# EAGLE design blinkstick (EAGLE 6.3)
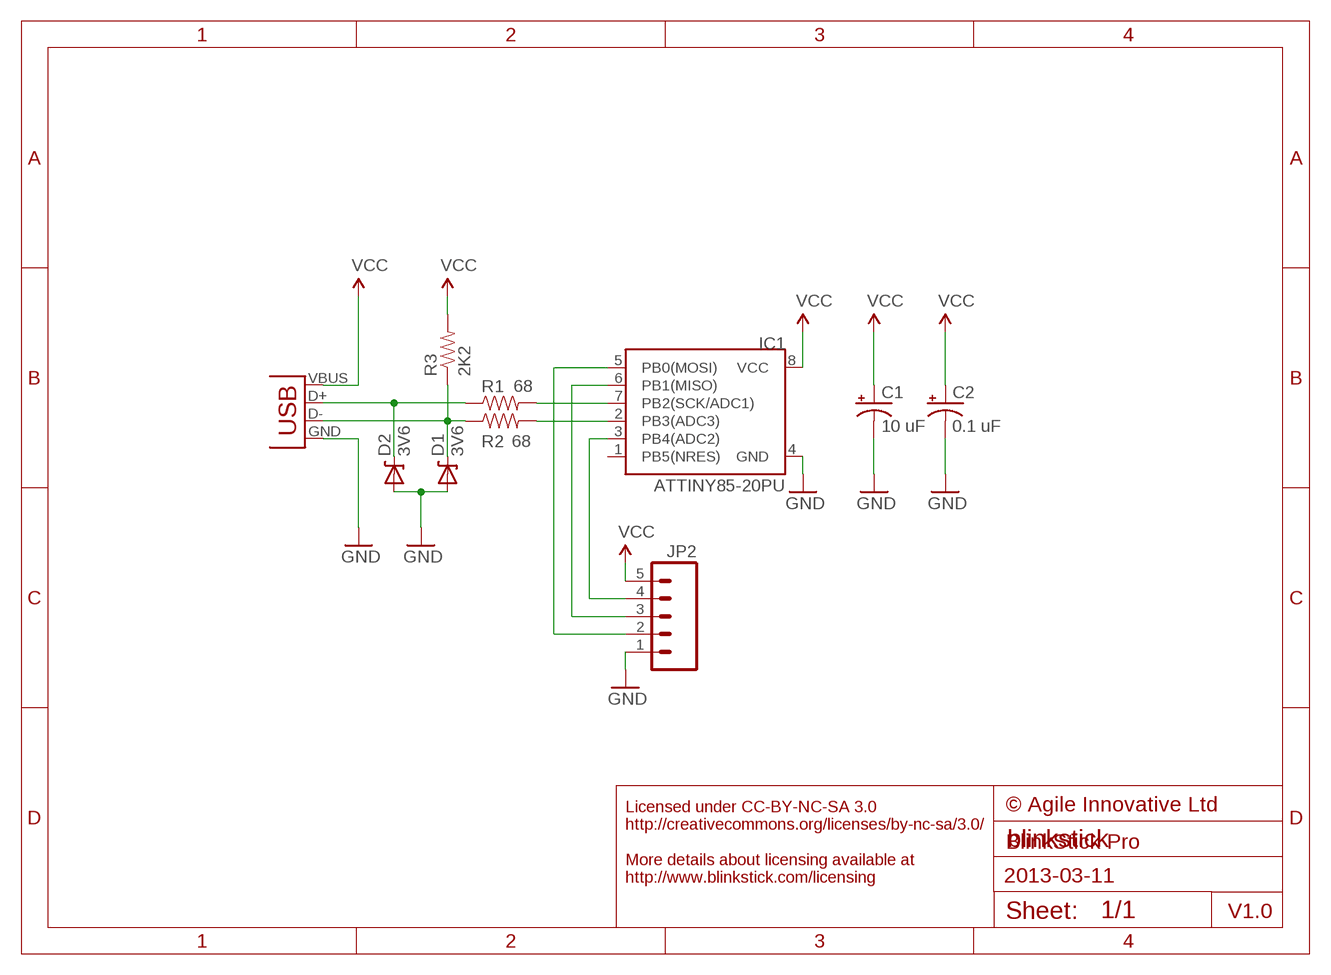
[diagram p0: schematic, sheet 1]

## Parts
C1  10 uF  CAP_POLPTH2  [CPOL-RADIAL-10UF-25V]
C2  0.1 uF  CAP_POLPTH2-1  [CPOL-PTH-10UF-25V]
D1  3V6  DIODE-ZENERPTH  [DIODE-ZENER]
D2  3V6  DIODE-ZENERPTH  [DIODE-ZENER]
IC1  ATTINY85-20PU  ATTINY45TINY45-20-DIP  [DIP08]
JP1  USB-A-H  [USB-A-H]
JP2  M05PTH  [1X05]
R1  68  RESISTORPTH-1/4W  [AXIAL-0.4]
R2  68  RESISTORPTH-1/4W  [AXIAL-0.4]
R3  2K2  RESISTORPTH-1/4W  [AXIAL-0.4]

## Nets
GND: C1.2(-) C2.2(-) D1.P$2(A) D2.P$2(A) IC1.4(GND) JP1.GND(VBUS) JP2.1
N$1: D2.P$1(C) JP1.D+(D-) R1.P$1
N$2: IC1.7(PB2(SCK/ADC1)) R1.P$2
N$3: IC1.2(PB3(ADC3)) R2.P$2
N$4: D1.P$1(C) JP1.D-(D+) R2.P$1 R3.P$1
N$5: IC1.3(PB4(ADC2)) JP2.4
N$6: IC1.6(PB1(MISO)) JP2.3
N$7: IC1.5(PB0(MOSI)) JP2.2
VCC: C1.1(+) C2.1(+) IC1.8(VCC) JP1.VBUS(GND) JP2.5 R3.P$2
Unconnected: IC1.1(PB5(NRES))

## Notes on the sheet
- © Agile Innovative Ltd
- BlinkStick Pro
- Licensed under CC-BY-NC-SA 3.0
  http://creativecommons.org/licenses/by-nc-sa/3.0/
  
  More details about licensing available at
  http://www.blinkstick.com/licensing
- 2013-03-11
- V1.0

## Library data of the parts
C1 = SparkFun-Capacitors:CAP_POL: Capacitor Polarized
C2 = generic:CAP_POL: Capacitor Polarized
D1 D2 = generic:DIODE-ZENER: Zener Diode
IC1 = SparkFun-DigitalIC big pads:ATTINY45: Atmel 8-pin 2/4/8kB flash uC; PROD_ID: IC-09439; VALUE: TINY45-20-DIP
JP1 = generic:USB: USB Connectors USB-B-PTH is fully proven SKU : PRT-00139/CONN-08278 USB-miniB is fully proven SKU : PRT-00587 USB-A-PCB is untested. USB-A-H is throughly reviewed, but untested. Spark Fun Electronics SKU : PRT-00437 USB-B-SMT is throughly reviewed, but untested. Needs silkscreen touching up.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
JP2 = SparkFun-Connectors:M05: Header 5 Standard 5-pin 0.1" header. Use with straight break away headers (SKU : PRT-00116), right angle break away headers (PRT-00553), swiss pins (PRT-00743), machine pins (PRT-00117), and female headers (PRT-00115). Molex polarized connector foot print use with SKU : PRT-08230 with associated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
R1-R3 = SparkFun-Passives:RESISTOR: Resistor

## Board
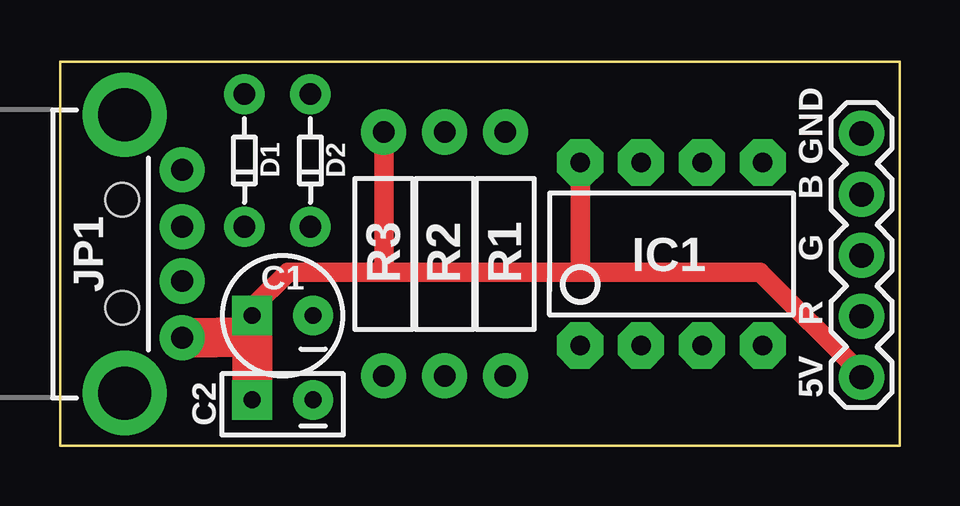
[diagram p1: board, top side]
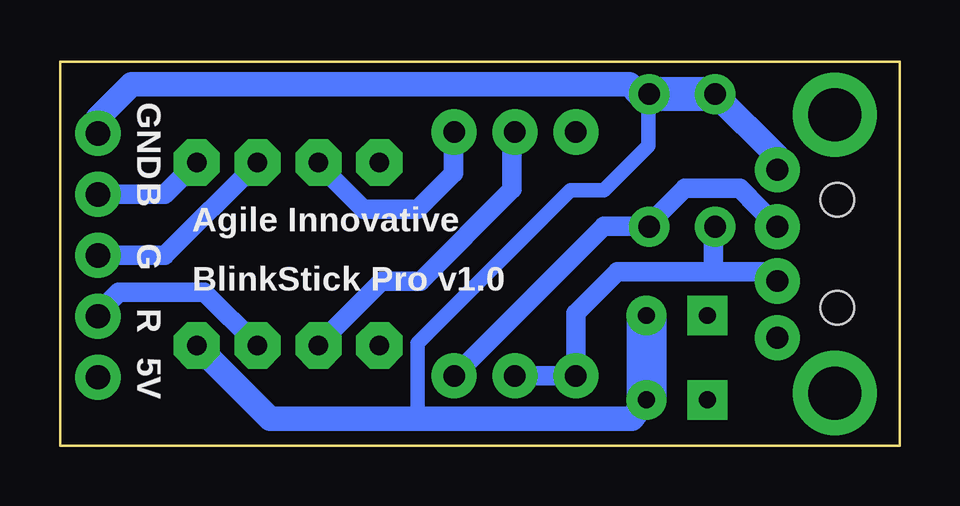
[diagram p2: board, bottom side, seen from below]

Size 35 x 16 mm. Coordinates in mm from the lower left corner, seen from the top.
Outline: 0,0 35,0 35,16 0,16 0,0
Copper layers (1*16): Top 0.035mm / dielectric 1.5mm / Bottom 0.035mm
Design rules "PCB-POOL Standard *": minimum track width 0.15mm, minimum drill 0.3mm, track to track 0.15mm, track to pad 0.15mm, pad to pad 0.15mm, via to via 0.15mm, smd to smd 0.15mm, copper to edge 0.3mm, drill to drill 0.2mm, minimum pad ring 0.2mm, minimum via ring 0.15mm, stop-mask expansion 0.075mm, vias tented up to drill 25mm, thermal gap 0.2mm

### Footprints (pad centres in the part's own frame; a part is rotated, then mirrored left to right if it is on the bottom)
CPOL-RADIAL-10UF-25V = drill 0.7 pad 1.651 square: 1 1.27,0 | drill 0.7 pad 1.651: 2 -1.27,0
CPOL-PTH-10UF-25V = drill 0.7 pad 1.651 square: 1 1.27,0 | drill 0.7 pad 1.651: 2 -1.27,0
DIODE-ZENER = drill 0.9 pad 1.676: P$1 -3.556,0; P$2 1.968,0
DIP08 = drill 0.813 pad 1.93 octagon: 1 -3.81,-3.81; 2 -1.27,-3.81; 3 1.27,-3.81; 4 3.81,-3.81; 5 3.81,3.81; 6 1.27,3.81; 7 -1.27,3.81; 8 -3.81,3.81
USB-A-H = drill 0.914 pad 1.88: D+ 2.4,1.127; D- 2.4,-1.127; GND 2.4,3.5; VBUS 2.4,-3.5 | drill 2.2: GND2 0,-5.8; GND3 0,5.8 | hole 1.4: -0.1,2.25; -0.1,-2.25
1X05 = drill 1.016 pad 1.88: 1 0,0; 2 2.54,0; 3 5.08,0; 4 7.62,0; 5 10.16,0
AXIAL-0.4 = drill 0.9 pad 1.88: P$1 -5.08,0; P$2 5.08,0

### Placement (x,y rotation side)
C1  9.28,5.43 180 top
C2  9.28,1.92 180 top
D1  7.69,12.69 90 top
D2  10.44,12.69 90 top
IC1  25.49,8 0 top
JP1  2.7,8 0 top
JP2  33.42,13.02 270 top
R1  18.57,8 90 top
R2  16.04,8 90 top
R3  13.49,8 90 top

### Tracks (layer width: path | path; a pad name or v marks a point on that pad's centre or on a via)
GND
  Bottom 0.61: 10.47,14.63 10.47,12.51 12.32,10.66 13.71,10.66 20.1,4.27 20.1,1.13
  Bottom 0.813: 10.47,14.63 D2.P$2 10.87,14.66 | D1.P$2
  Bottom 1.016: C2.2 11.15,1.13 20.1,1.13 26.24,1.13 IC1.4 | JP1.GND 5.1,12.07 D1.P$2 | 10.87,14.66 11.27,15.06 32.02,15.06 33.42,13.66 JP2.1
  Bottom 1.422: D1.P$2 D2.P$2
  Bottom 1.676: C1.2 C2.2
N$1
  Bottom 0.813: JP1.D+ 6.66,10.74 8.94,10.74 10.44,9.23 D2.P$1 10.47,9.11 10.51,9.14 12.33,9.14 18.55,2.92 R1.P$1
N$2
  Bottom 0.813: IC1.7 24.22,11.74 22.35,9.87 20.09,9.87 18.59,11.37 18.59,13.06 R1.P$2
N$3
  Bottom 0.406: R2.P$2 16.16,12.96 | 24.22,4.24 IC1.2
  Bottom 0.813: 16.16,12.96 16.16,10.69 19.98,6.87 21.59,6.87 24.22,4.24
N$4
  Bottom 0.813: R2.P$1 R3.P$1 13.49,5.52 11.75,7.26 7.75,7.26 | 7.75,7.26 5.43,7.26 JP1.D- | D1.P$1 7.75,9.13 7.75,7.26
N$5
  Bottom 0.813: IC1.3 28.98,6.41 32.55,6.41 33.42,5.54 JP2.4
N$6
  Bottom 0.813: IC1.6 30.63,7.94 JP2.3
N$7
  Bottom 0.813: IC1.5 30.63,10.48 JP2.2
VCC
  Top 0.813: 7.99,4.55 8.01,4.58 | 8.01,5.75 9.5,7.24 13.52,7.24 | 13.52,7.24 21.7,7.24 | 13.52,13.08 13.52,7.24 | 21.7,11.81 21.7,7.24 | 21.7,7.24 29.18,7.24 33.42,3 JP2.5
  Top 1.016: 8.01,4.58 C1.1 8.01,5.75 | R3.P$2 13.52,13.08 | IC1.8 21.7,11.81
  Top 1.676: 8.01,4.58 C2.1 | JP1.VBUS 7.99,4.55

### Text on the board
tNames: GND | B | G | R | 5V | 5V
bNames: GND | B | Agile Innovative | G | BlinkStick Pro v1.0 | R | 5V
